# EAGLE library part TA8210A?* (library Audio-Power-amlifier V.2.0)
20W BTL × 2ch Audio Power Amplifier Source: http://www.semicon.toshiba.co.jp/td/en/ASSP/Audio_ICs/en_20050517_TA8210ALQ_datasheet.pdf
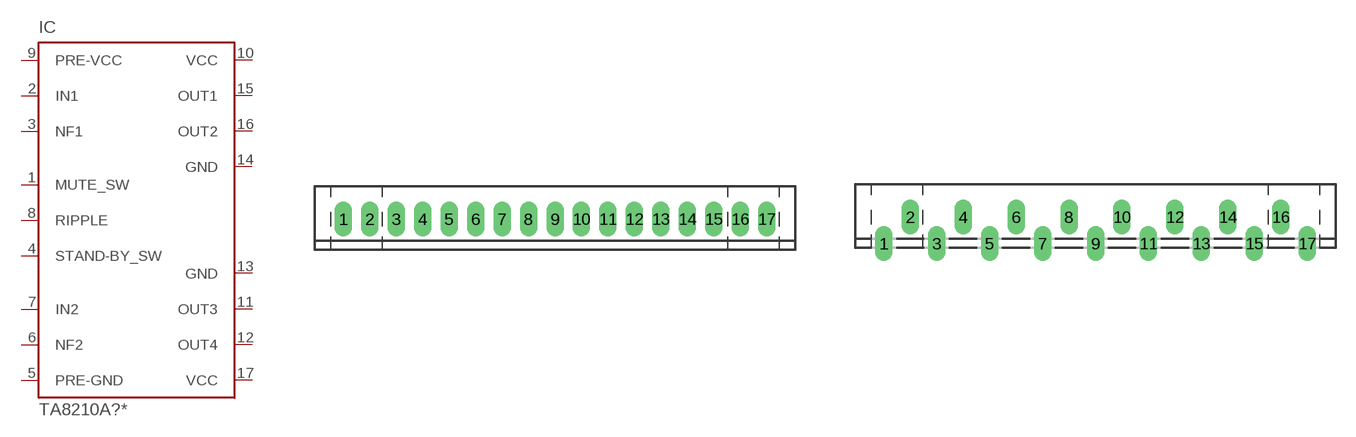
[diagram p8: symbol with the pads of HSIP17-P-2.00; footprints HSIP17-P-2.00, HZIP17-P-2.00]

Designator prefix IC

## TA8210AL, TA8210ALQ  [HSIP17-P-2.00]
1  MUTE_SW  in
2  IN1  in
3  NF1  in
4  STAND-BY_SW  in
5  PRE-GND  pwr
6  NF2  in
7  IN2  in
8  RIPPLE  in
9  PRE-VCC  pwr
10  VCC  pwr
11  OUT3  out
12  OUT4  out
13  GND  pwr
14  GND  pwr
15  OUT1  out
16  OUT2  out
17  VCC  pwr

## TA8210AH, TA8210AHQ  [HZIP17-P-2.00]
Pads as for HSIP17-P-2.00

## Footprint HSIP17-P-2.00 (pad centres in mm)
HSIP17-P-2.00 Source: http://www.semicon.toshiba.co.jp/td/en/ASSP/Audio_ICs/en_20050517_TA8210ALQ_datasheet.pdf
drill 0.8 pad 1.2 long: 1 -16,0; 2 -14,0; 3 -12,0; 4 -10,0; 5 -8,0; 6 -6,0; 7 -4,0; 8 -2,0; 9 0,0; 10 2,0; 11 4,0; 12 6,0; 13 8,0; 14 10,0; 15 12,0; 16 14,0; 17 16,0

## Footprint HZIP17-P-2.00 (pad centres in mm)
HZIP17-P-2.00 Source: http://www.semicon.toshiba.co.jp/td/en/ASSP/Audio_ICs/en_20050517_TA8210ALQ_datasheet.pdf
drill 0.8 pad 1.2 long: 1 -16,-2; 2 -14,0; 3 -12,-2; 4 -10,0; 5 -8,-2; 6 -6,0; 7 -4,-2; 8 -2,0; 9 0,-2; 10 2,0; 11 4,-2; 12 6,0; 13 8,-2; 14 10,0; 15 12,-2; 16 14,0; 17 16,-2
